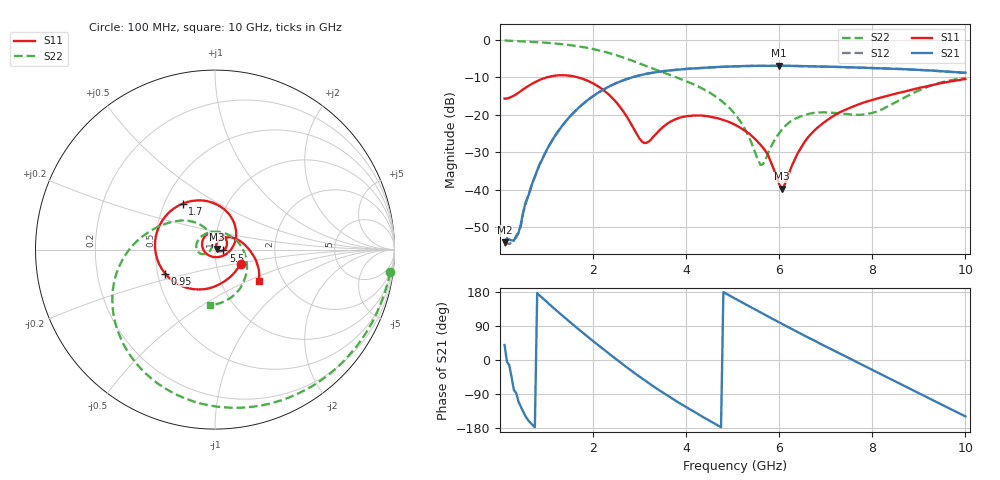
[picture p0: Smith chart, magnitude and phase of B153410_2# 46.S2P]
!  2-Port S-parameters saved by WinCal
! VAR MeasName=S-Parameters (CALIBRATED_DATA) read from VNA (N5245A)
! VAR MeasDate=2016-12-23 10:01:44
! VAR NAME=B153410_2# 46
! VAR FILENAME=B153410_2# 46.S2P
! VAR DATE=2016-12-23 10:01:44
! VAR PHYS_PORTS=1,2
# Hz S DB R 50
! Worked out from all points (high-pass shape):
!   199 points, 100 MHz to 10 GHz, reference 50 ohm
!   highest |S21| = -6.88 dB at 6 GHz (marker M1); lowest = -54.1 dB at 100 MHz (marker M2)
!   |S21| within 3 dB of the highest: 2.874 GHz to end of sweep
!   lowest |S11| = -39.7 dB at 6.05 GHz (marker M3), VSWR 1.02, Z = 51 + j0.391 ohm
!   |S11| at or under -10 dB: start of sweep to 1.009 GHz; 1.675 GHz to end of sweep
!   |S22| runs from -33.4 to -0.1 dB; largest |S21 - S12| = 0.004
!   S11 on the Smith chart (normalised r, x): 100 MHz: 1.32, -0.21; 950 MHz: 0.55, -0.16; 1.7 GHz: 0.62, +0.35; 5.5 GHz: 1.10, -0.01; 10 GHz: 1.51, -0.58
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1e8  -15.67 -28.6  -54.05 39.6  -55.14 32.3  -0.13 -7.4
4e8  -14.09 -84.7  -51.50 -110.8  -51.56 -110.6  -0.33 -27.6
5.5e8  -12.78 -105.8  -43.44 -148.7  -44.13 -148.9  -0.43 -37.5
9.5e8  -10.24 -154.1  -30.75 159.4  -30.83 159.7  -0.71 -63.5
1.3e9  -9.43 167.3  -23.56 121.5  -23.55 121.4  -1.09 -85.8
1.7e9  -10.08 125.0  -18.00 80.0  -18.04 80.0  -1.73 -110.6
1.75e9  -10.28 119.8  -17.47 75.1  -17.49 75.0  -1.83 -113.6
2.4e9  -15.33 48.7  -12.10 11.3  -12.10 11.4  -3.69 -150.8
3.1e9  -27.57 -90.9  -9.17 -52.7  -9.17 -52.7  -6.77 177.1
3.4e9  -24.49 -169.9  -8.53 -77.9  -8.51 -77.9  -8.18 166.4
4.15e9  -20.19 102.1  -7.59 -135.2  -7.61 -135.2  -11.80 141.3
5.05e9  -22.69 24.9  -7.04 162.1  -7.05 162.2  -19.81 109.3
5.5e9  -26.69 -5.9  -6.92 132.0  -6.92 132.0  -30.67 120.1
5.65e9  -28.77 -13.4  -6.93 122.0  -6.91 122.1  -33.26 167.8
6e9  -38.60 3.4  -6.88 99.3  -6.89 99.4  -24.90 -154.8
6.05e9  -39.74 21.8  -6.90 96.1  -6.91 96.1  -24.11 -156.6
6.4e9  -30.22 75.1  -6.95 73.5  -6.96 73.6  -20.76 -170.1
6.7e9  -24.92 65.8  -7.01 54.5  -7.03 54.5  -19.60 173.4
7.5e9  -18.23 31.7  -7.28 4.9  -7.31 4.9  -19.90 114.3
8.35e9  -14.81 3.6  -7.66 -47.5  -7.66 -47.3  -17.64 21.6
9.15e9  -12.44 -15.6  -8.08 -96.7  -8.11 -96.6  -12.74 -43.6
1e10  -10.45 -35.6  -8.78 -148.8  -8.80 -148.2  -10.18 -95.4
